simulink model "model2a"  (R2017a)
settings: Solver=ode5  StartTime=0.0  StopTime=100  FixedStep=0.1  RelTol=1e-3
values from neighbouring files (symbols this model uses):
  dist_t = 1    [Mandatory2a.m]    (also in Mandatory2b.m = 10; Mandatory2c.m = 10)
  dist_val = 1    [Mandatory2a.m]    (also in Mandatory2b.m; Mandatory2c.m)
  K = 5    [Mandatory2a.m]    (also in Mandatory2b.m; Mandatory2c.m)
  SetPoint = 0    [Mandatory2a.m]    (also in Mandatory2b.m; Mandatory2c.m)
  T = 10    [Mandatory2a.m]    (also in Mandatory2b.m; Mandatory2c.m)
  tau = 2    [Mandatory2a.m]    (also in Mandatory2b.m; Mandatory2c.m)
libraries: simulink x1

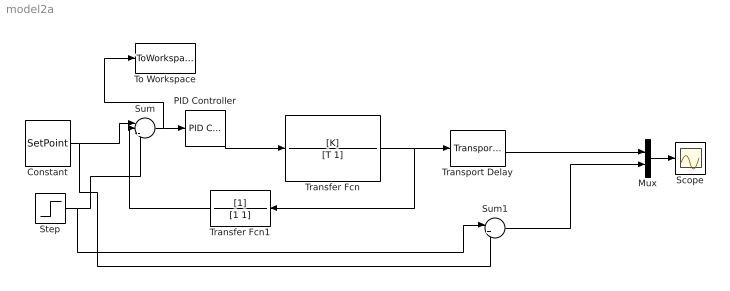
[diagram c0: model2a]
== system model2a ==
  Constant : Constant  Value=SetPoint
  Mux : Mux  Inputs=2
  PID Controller : simulink/Continuous/PID Controller  Controller=PID  TimeDomain=Continuous-time  SampleTime=-1  IntegratorMethod=Forward Euler  FilterMethod=Forward Euler  Form=Parallel  UseFilter=on  ControllerParametersSource=internal  P=2  I=1  D=0  N=100  InitialConditionSource=internal  InitialConditionForIntegrator=0  InitialConditionForFilter=0  ExternalReset=none  LimitOutput=off  UpperSaturationLimit=inf  LowerSaturationLimit=-inf  LinearizeAsGain=on  AntiWindupMode=none  Kb=1  TrackingMode=off  Kt=1  PParamMin=[]  PParamMax=[]  IParamMin=[]  IParamMax=[]  DParamMin=[]  DParamMax=[]  NParamMin=[]  NParamMax=[]  KbParamMin=[]  KbParamMax=[]  KtParamMin=[]  KtParamMax=[]  POutMin=[]  POutMax=[]  IOutMin=[]  IOutMax=[]  DOutMin=[]  DOutMax=[]  NOutMin=[]  NOutMax=[]  KbOutMin=[]  KbOutMax=[]  KtOutMin=[]  KtOutMax=[]  IntegratorOutMin=[]  IntegratorOutMax=[]  FilterOutMin=[]  FilterOutMax=[]  SumOutMin=[]  SumOutMax=[]  SumI1OutMin=[]  SumI1OutMax=[]  SumI2OutMin=[]  SumI2OutMax=[]  SumI3OutMin=[]  SumI3OutMax=[]  SumDOutMin=[]  SumDOutMax=[]  SaturationOutMin=[]  SaturationOutMax=[]  IntegratorContinuousStateAttributes=''  IntegratorStateMustResolveToSignalObject=off  IntegratorRTWStateStorageClass=Auto  FilterContinuousStateAttributes=''  FilterStateMustResolveToSignalObject=off  FilterRTWStateStorageClass=Auto  DifferentiatorICPrevScaledInput=0  DifferentiatorOutMin=[]  DifferentiatorOutMax=[]  InitialConditionSetting=State (most efficient)
  Scope : Scope
  Step : Step  Time=dist_t  After=dist_val  SampleTime=0
  Sum : Sum  Inputs=|+-+
  Sum1 : Sum  Inputs=|++
  To Workspace : ToWorkspace  VariableName=d_error  SampleTime=-1
  Transfer Fcn : TransferFcn  Numerator=[K]  Denominator=[T 1]
  Transfer Fcn1 : TransferFcn  Denominator=[1 1]
  Transport Delay : TransportDelay  DelayTime=tau
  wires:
  Transfer Fcn/1 -> Transfer Fcn1/1, Transport Delay/1
  Step/1 -> Sum1/1, Sum/3
  Sum/1 -> To Workspace/1, PID Controller/1
  Mux/1 -> Scope/1
  Transport Delay/1 -> Mux/1
  Transfer Fcn1/1 -> Sum/2
  Constant/1 -> Sum1/2, Sum/1
  PID Controller/1 -> Transfer Fcn/1
  Sum1/1 -> Mux/2
